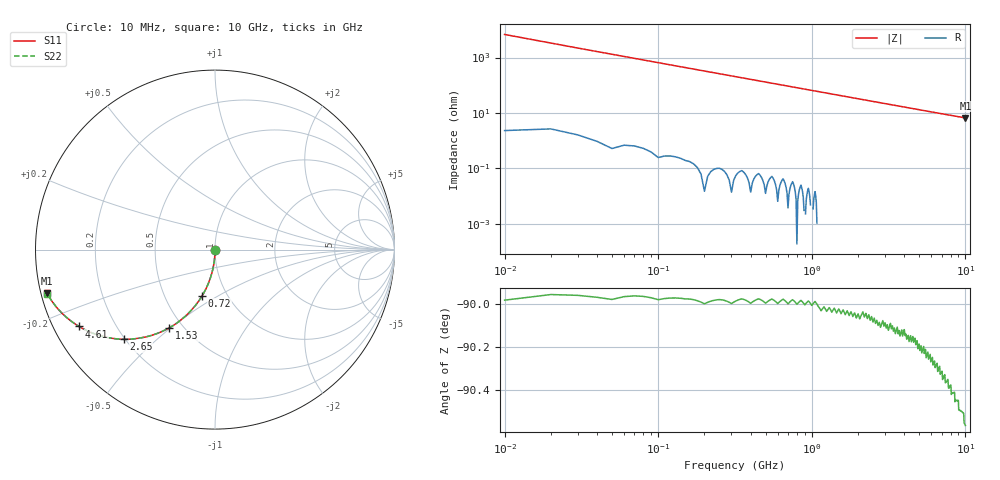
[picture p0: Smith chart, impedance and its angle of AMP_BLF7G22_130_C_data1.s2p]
! Created Thu Jul 08 13:17:30 2010
# ghz S ma R 50
! 2 Port Network Data from SP1.SP block
! freq  magS11  angS11  magS21  angS21  magS12  angS12  magS22  angS22
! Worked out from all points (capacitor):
!   1000 points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, 10 MHz to 10 GHz, reference 50 ohm
!   read as one part in shunt: C = 2.45 pF near 60 MHz
!   lowest |Z| = 6.61 ohm at 10 GHz (marker M1)
!   S11 on the Smith chart (normalised r, x): 10 MHz: 1.00, -0.01; 720 MHz: 0.77, -0.42; 1.53 GHz: 0.42, -0.49; 2.65 GHz: 0.19, -0.40; 4.61 GHz: 0.07, -0.26; 10 GHz: 0.02, -0.13
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0.01  0.003601 -89.9  1 -0.2  1 -0.2  0.0037 -89.9
0.04  0.01484 -90.8  0.9998 -0.9  0.9998 -0.9  0.0154 -90.8
0.07  0.02655 -91.5  0.9996 -1.5  0.9996 -1.5  0.02697 -91.5
0.09  0.03451 -92.0  0.9993 -2.0  0.9993 -2.0  0.03464 -92.0
0.11  0.04217 -92.4  0.999 -2.4  0.999 -2.4  0.0423 -92.4
0.14  0.05323 -93.1  0.9985 -3.1  0.9985 -3.1  0.05376 -93.1
0.2  0.07665 -94.4  0.997 -4.4  0.997 -4.4  0.07658 -94.4
0.29  0.1106 -96.4  0.9938 -6.4  0.9938 -6.4  0.1107 -96.4
0.41  0.1556 -99.0  0.9877 -9.0  0.9877 -9.0  0.1556 -99.0
0.55  0.2061 -102.0  0.9783 -12.0  0.9783 -12.0  0.2067 -101.9
0.72  0.2663 -105.5  0.9637 -15.5  0.9637 -15.5  0.2665 -105.5
1.1  0.3891 -112.9  0.921 -23.0  0.921 -23.0  0.3891 -112.9
1.53  0.5068 -120.4  0.8621 -30.5  0.8621 -30.5  0.5063 -120.5
1.68  0.5422 -122.8  0.8403 -32.9  0.8403 -32.9  0.5418 -122.8
2.13  0.6327 -129.3  0.7742 -39.4  0.7742 -39.4  0.6327 -129.3
2.65  0.7129 -135.5  0.7014 -45.6  0.7014 -45.6  0.7127 -135.5
3.34  0.7882 -142.1  0.6158 -52.2  0.6158 -52.2  0.788 -142.0
4.61  0.8705 -150.6  0.4935 -60.7  0.4935 -60.7  0.8699 -150.5
5.01  0.8869 -152.6  0.4629 -62.8  0.4629 -62.8  0.8867 -152.5
6.67  0.9313 -158.7  0.3664 -69.0  0.3664 -69.0  0.9308 -158.6
8.34  0.9542 -162.7  0.3015 -73.1  0.3015 -73.1  0.9539 -162.6
10  0.9675 -165.4  0.2561 -76.0  0.2561 -76.0  0.9672 -165.3
